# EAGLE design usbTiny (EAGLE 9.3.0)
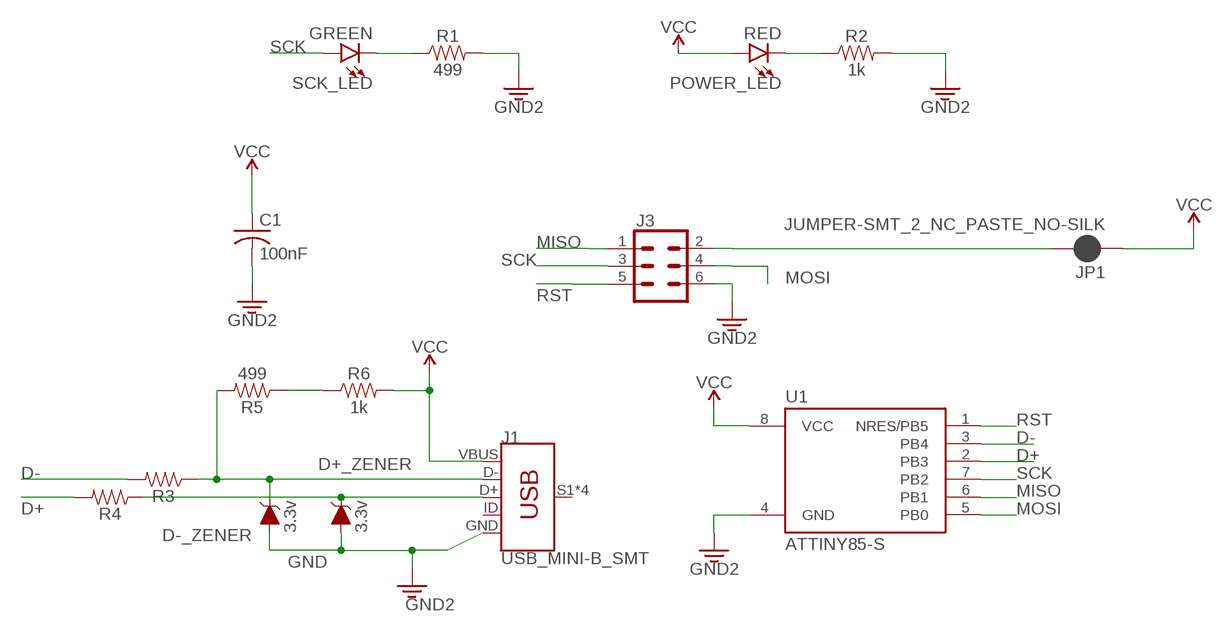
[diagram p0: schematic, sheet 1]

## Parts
C1  100nF  C-USC1206K  [C1206K]
D+_ZENER  3.3v  DIODE-ZENER-DZ2J150M0L  [PANASONIC_SMINI2-F5-B]
D-_ZENER  3.3v  DIODE-ZENER-DZ2J150M0L  [PANASONIC_SMINI2-F5-B]
J1  USB_MINI-B_SMT  [USB-MINIB]
J3  CONN_03X2FEMALE_SMD  [2X3_SMD]
JP1  JUMPER-SMT_2_NC_PASTE_NO-SILK  [SMT-JUMPER_2_NC_PASTE_NO-SILK]
POWER_LED  RED  LED-RED1206  [LED-1206]
R1  499  RESISTOR1206  [1206]
R2  1k  RESISTOR1206  [1206]
R3  RESISTOR1206  [1206]
R4  RESISTOR1206  [1206]
R5  499  RESISTOR1206  [1206]
R6  1k  RESISTOR1206  [1206]
SCK_LED  GREEN  LED-GREEN1206  [LED-1206]
U1  ATTINY85-S  [SOIC8_EIAJ_208MIL]

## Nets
3.3V: U1.4(GND) ; supply symbol labelled GND2
D+: R4.2 U1.2(PB3)
D-: R3.2 U1.3(PB4)
GND: C1.2 D+_ZENER.A D-_ZENER.A J1.GND J3.6 R1.2 R2.2 ; supply symbol labelled GND2
MISO: J3.1 U1.6(PB1)
MOSI: J3.4 U1.5(PB0)
N$1: R1.1 SCK_LED.C
N$2: POWER_LED.C R2.1
N$3: D+_ZENER.C J1.D+ R4.1
N$4: D-_ZENER.C J1.D- R3.1 R5.2
N$5: R5.1 R6.1
N$6: J3.2 JP1.2
RST: J3.5 U1.1(NRES/PB5)
SCK: J3.3 SCK_LED.A U1.7(PB2)
VCC: C1.1 J1.VBUS JP1.1 POWER_LED.A R6.2 U1.8(VCC)
Unconnected: J1.ID J1.S1(SHIELD) J1.S2(SHIELD) J1.S3(SHIELD) J1.S4(SHIELD)

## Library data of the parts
C1 = adafruit:C-US: CAPACITOR, American symbol
D+_ZENER D-_ZENER = SparkFun-DiscreteSemi:DIODE-ZENER: Zener Diode; PROD_ID: DIO-12989; VALUE: 15V
J1 = SparkFun-Connectors:USB_MINI-B: USB type Mini-B Connector Breaks out 5th pin, and includes shield pins if needed. SparkFun Products: SparkFun FTDI Basic Breakout SparkFun XBee Explorer USB SparkFun Redboard; PROD_ID: CONN-08193; SF_ID: PRT-00587
J3 = SparkFun-Connectors:CONN_03X2: Multi connection point. Often used as Generic Header-pin footprint for 0.1 inch spaced/style header connections You can populate with any combo of single row headers, but if you'd like an exact match, check these: Header - 2x3 (Male, 0.1") (PRT-12807) Header - 2x3 (Female, 0.1") (PRT-13010) 2x3 Pin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; PROD_ID: CONN-11290
JP1 = SparkFun-Jumpers:JUMPER-SMT_2_NC_PASTE: Normally closed solder jumper
POWER_LED = SparkFun-LED:LED-RED: Red SMD LED; PROD_ID: DIO-09912
R1-R6 = SparkFun-Resistors:RESISTOR: Generic Resistor Package
SCK_LED = SparkFun-LED:LED-GREEN: Green SMD LED; PROD_ID: DIO-00862
U1 = _hhn_attiny25_45_85:ATTINY85*: ATMEL ATtiny 85 Packages: P = PDIP 08 30mil S = SOIC 08 EIAJ 208mil Technologies Note: for complete ordering code (temp. range, finish, tape&reel etc.) see www.atmel.com &bull; Supply Voltage: V = (1.8&hellip;5.5)V | [blank] = (2.7&hellip;5.5)V &bull; Speed: 10 = 10 MHz | 20 = 20 MHz Author: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

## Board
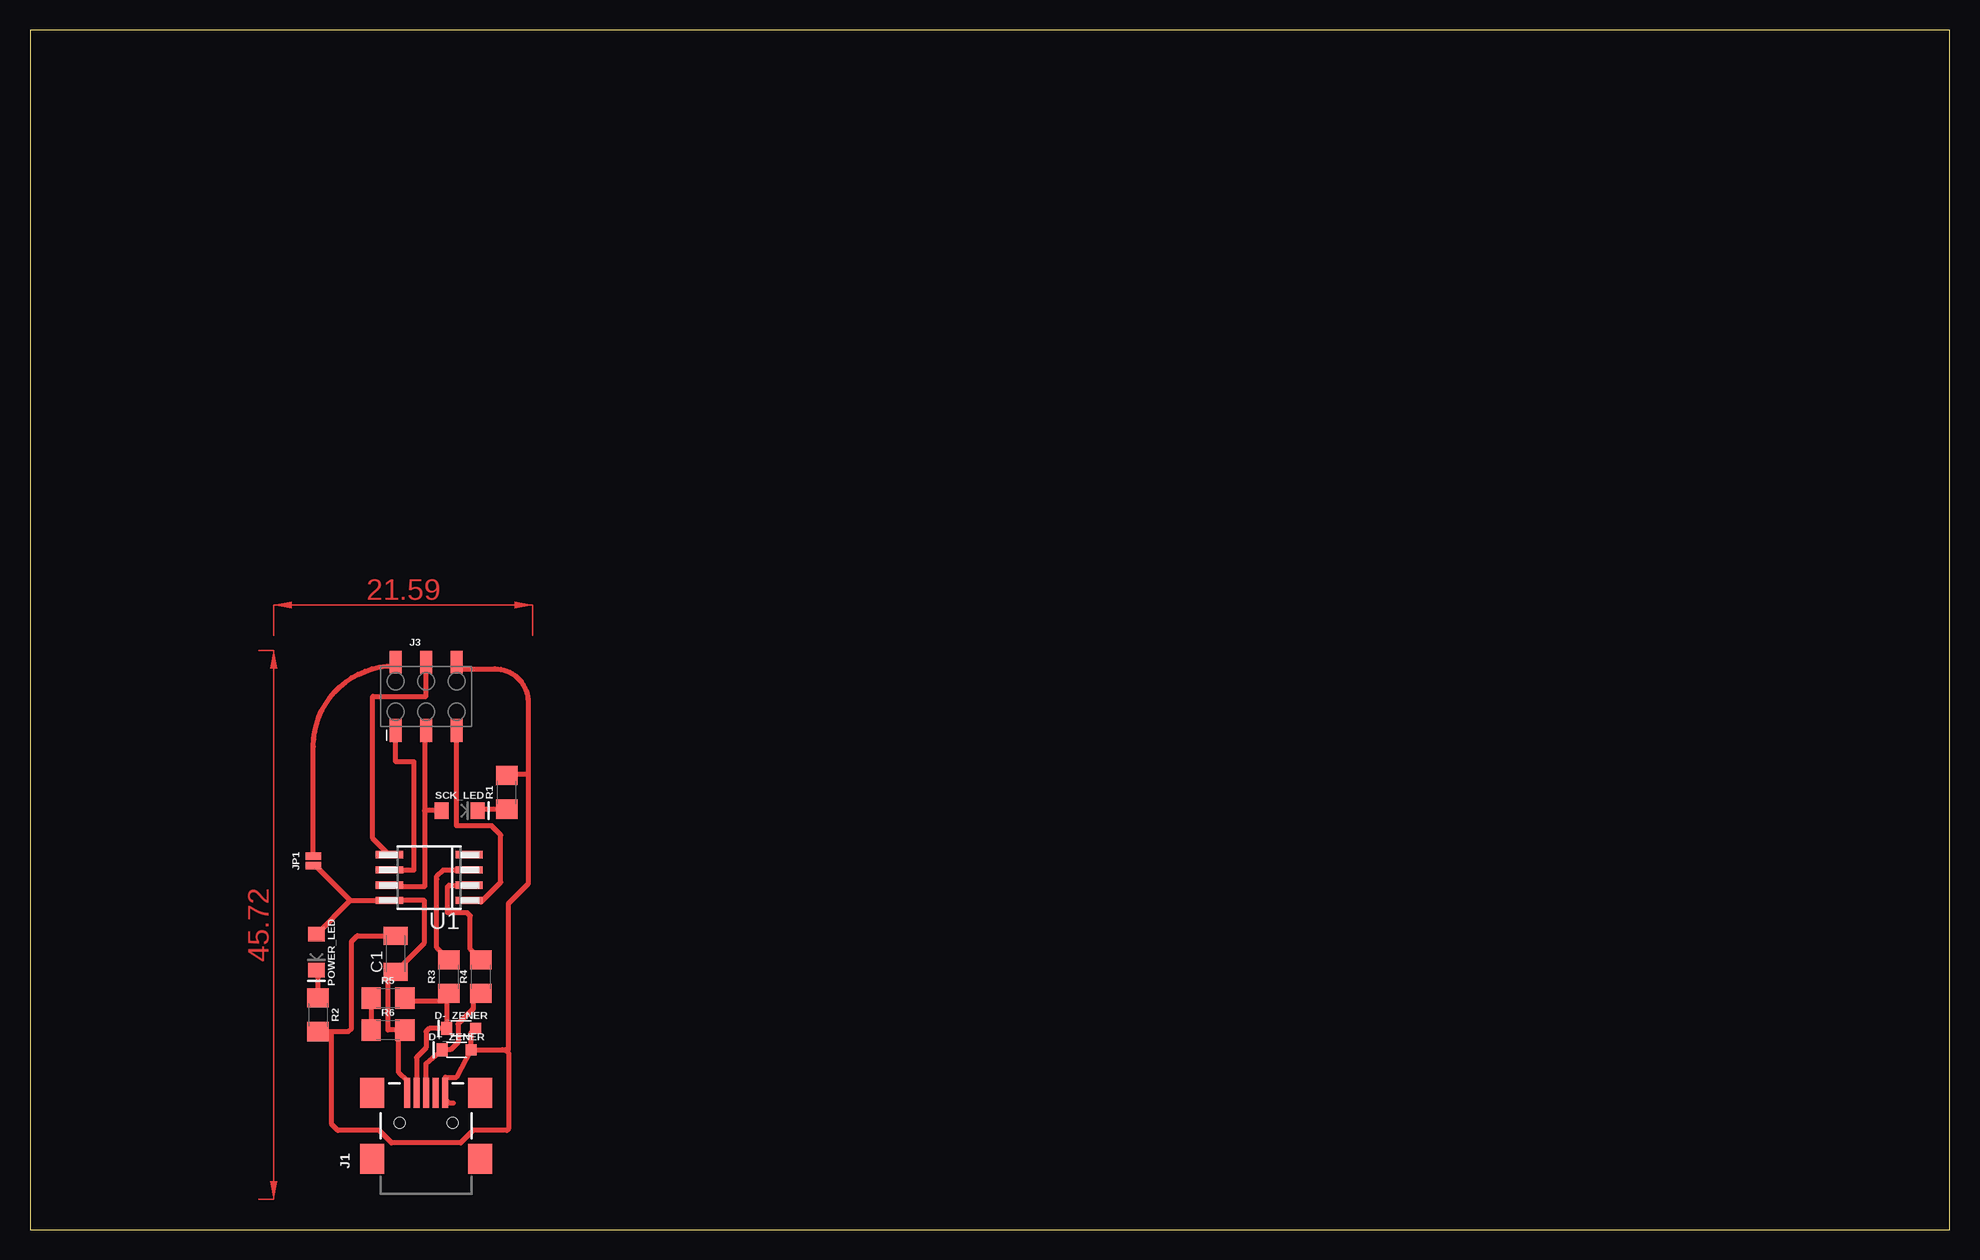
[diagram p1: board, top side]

Size 160 x 100 mm. Coordinates in mm from the lower left corner, seen from the top.
Outline: 0,0 160,0 160,100 0,100 0,0
Copper layers (1*16): Top 0.035mm / dielectric 1.5mm / Bottom 0.035mm
Design rules "default": minimum track width 6mil, minimum drill 0.35mm, track to track 6mil, track to pad 6mil, pad to pad 6mil, via to via 6mil, smd to smd 6mil, copper to edge 40mil, drill to drill 6mil, minimum pad ring 10mil, minimum via ring 8mil, stop-mask expansion 4mil, vias tented up to drill 0mil, thermal gap 10mil

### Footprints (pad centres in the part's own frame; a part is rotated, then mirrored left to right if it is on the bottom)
C1206K = smd 1.5 x 2: 1 -1.5,0; 2 1.5,0
PANASONIC_SMINI2-F5-B = smd 0.9 x 0.9: A 1.2,0 | smd 0.9 x 1.1: C -1.2,0
USB-MINIB = smd 2.5 x 0.5: D+ 2.5,0; D- 2.5,0.8; GND 2.5,-1.6; ID 2.5,-0.8; VBUS 2.5,1.6 | smd 2.5 x 2: S1 -3,4.5; S2 2.5,4.5; S3 -3,-4.5; S4 2.5,-4.5 | hole 0.9: 0,2.2; 0,-2.2
2X3_SMD = smd 1.02 x 1.9: 1 -2.54,-2.85; 2 -2.54,2.85; 3 0,-2.85; 4 0,2.85; 5 2.54,-2.85; 6 2.54,2.85
SMT-JUMPER_2_NC_PASTE_NO-SILK = smd 0.635 x 1.27: 1 -0.406,0; 2 0.406,0
LED-1206 = smd 1.2 x 1.4: A -1.5,0; C 1.5,0
1206 = smd 1.6 x 1.8: 1 -1.4,0; 2 1.4,0
SOIC8_EIAJ_208MIL = smd 0.6 x 2.286: 1 -1.905,-3.33; 2 -0.635,-3.33; 3 0.635,-3.33; 4 1.905,-3.33; 5 1.905,3.33; 6 0.635,3.33; 7 -0.635,3.33; 8 -1.905,3.33

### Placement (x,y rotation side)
C1  30.48,22.99 90 top
D+_ZENER  35.56,14.99 0 top
D-_ZENER  35.94,16.76 0 top
J1  33.02,8.89 90 top
J3  33.02,44.45 0 top
JP1  23.62,30.73 90 top
POWER_LED  23.88,23.11 270 top
R1  39.75,36.45 90 top
R2  24,17.91 270 top
R3  34.92,21.08 90 top
R4  37.59,21.08 90 top
R5  29.84,19.3 0 top
R6  29.84,16.64 0 top
SCK_LED  35.81,34.92 0 top
U1  33.27,29.34 90 top

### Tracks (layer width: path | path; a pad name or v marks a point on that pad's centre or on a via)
D+
  Top 0.406: R4.2 36.7,23.37 36.7,26.16 36.45,26.42 34.8,26.42 34.8,28.57 34.92,28.7 U1.2
D-
  Top 0.406: R3.2 33.91,23.5 33.91,29.21 33.91,29.46 34.42,29.97 U1.3
GND
  Top 0.406: D+_ZENER.A 35.56,12.7 34.62,12.7 J1.GND 34.62,10.85 34.91,10.56 35.31,10.56 | D+_ZENER.A 36.76,16.38 D-_ZENER.A | R2.2 25.15,16.51 | 25.15,16.51 26.54,16.51 26.8,16.76 26.8,24 27.28,24.49 C1.2 | D+_ZENER.A 39.37,14.99 39.62,14.99 | 39.62,14.99 39.88,14.99 39.88,27.18 41.53,28.83 41.53,37.97 | 39.62,14.99 39.88,14.73 39.88,8.38 39.75,8.26 36.95,8.26 35.91,7.22 30.13,7.22 29.09,8.26 25.65,8.26 25.15,8.76 25.15,16.51 | J3.6 arc90 36.12,46.74 38.73,46.74 arc-90 41.53,43.94 41.53,37.97 | R1.2 39.75,37.97 41.53,37.97
MISO
  Top 0.406: U1.6 32,29.97 32,38.99 30.48,38.99 J3.1
MOSI
  Top 0.406: U1.5 28.57,32.61 28.57,44.45 33.02,44.45 J3.4
N$1
  Top 0.406: SCK_LED.C 37.31,35.05 R1.1
N$2
  Top 0.406: R2.1 24,21.49 POWER_LED.C
N$3
  Top 0.406: J1.D+ 33.02,13.84 D+_ZENER.C 35.05,14.99 35.69,15.62 35.69,17.14 36.96,18.41 36.96,19.68 R4.1
N$4
  Top 0.406: R3.1 34.74,19.5 34.74,19.05 | 34.74,19.05 D-_ZENER.C 33.27,16.76 33.02,16.51 33.02,15.15 32.22,14.35 J1.D- | R5.2 31.5,19.05 34.74,19.05
N$5
  Top 0.406: R5.1 R6.1
N$6
  Top 0.406: 30.35,46.99 30.35,47.17 arc-90 J3.2 30.48,46.74 | 30.35,46.99 30.35,46.61 | 30.48,46.74 arc-90 30.35,46.61 | 30.48,46.74 arc-90 30.35,46.61 | JP1.2 23.62,40.26 arc-90 30.35,46.99
RST
  Top 0.406: U1.1 37.47,27.43 37.59,27.3 39.24,28.96 39.24,32.89 38.48,33.66 36.83,33.66 36.7,33.66 35.56,33.66 J3.5
SCK
  Top 0.406: J3.3 32.89,41.6 32.89,34.92 | 32.89,34.92 32.89,28.57 30.48,28.57 30.48,28.83 29.94,28.83 U1.7 | SCK_LED.A 32.89,34.92
VCC  (2 unrouted)
  Top 0.406: R6.2 31.42,16.46 31.42,15.93 | C1.1 30.53,21.54 | 30.53,21.54 32.89,23.9 32.89,27.43 30.48,27.43 | POWER_LED.A 26.69,27.43 | 26.69,27.43 29.08,27.43 | 26.69,27.43 23.8,30.33 JP1.1 | J1.VBUS 31.42,12.39 30.73,13.08 30.73,16.13 30.74,16.13 R6.2 | R6.2 29.84,16.64 29.84,21.08 29.97,21.08 30.48,21.59 30.53,21.54
(copper drawn outside any net)
  shapes: Top area x2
